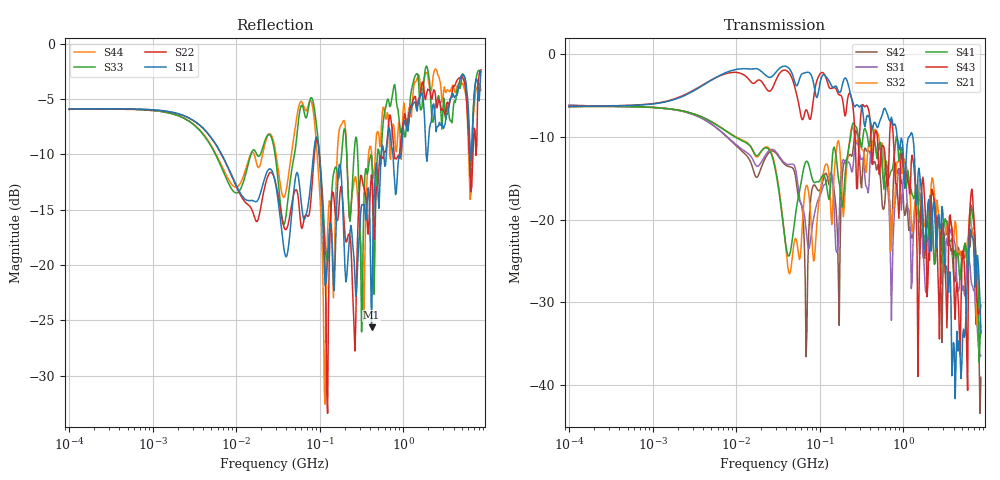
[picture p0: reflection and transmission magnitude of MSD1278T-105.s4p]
# MHz S MA R 50
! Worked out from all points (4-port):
!   498 points, 100 kHz to 8.5 GHz, reference 50 ohm
!   strongest paths, dB at 100 kHz, 1.698 MHz, 29.49 MHz, 500.7 MHz, 8.5 GHz:
!     S21: -6.3, -5.6, -2.3, -8.8, -33.7
!     S43: -6.3, -5.5, -3.3, -11.8, -30.4
!     S41: -6.4, -6.7, -14.0, -11.9, -33.4
!     S32: -6.4, -6.7, -13.7, -9.6, -32.9
!     S31: -6.2, -6.7, -11.7, -12.0, -36.4
!     S42: -6.2, -6.7, -11.9, -13.3, -39.1
!   lowest |S11| = -25.6 dB at 417.1 MHz (marker M1), VSWR 1.11, Z = 55.5 + j0.687 ohm
!   |S11| at or under -10 dB: 6.726 MHz to 84.3 MHz (77.58 MHz wide, 170 % of centre); 98.74 MHz to 546.1 MHz (447.3 MHz wide, 139 % of centre); 752.1 MHz to 938.7 MHz (186.6 MHz wide, 22.1 % of centre)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
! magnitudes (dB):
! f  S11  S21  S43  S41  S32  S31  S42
! 100 kHz  -5.9  -6.3  -6.3  -6.4  -6.4  -6.2  -6.2
! 68.65 MHz  -15.5  -2.2  -6.7  -13.0  -15.9  -21.2  -36.6
! 113.5 MHz  -20.3  -2.5  -2.4  -14.7  -13.8  -15.8  -14.7
! 417.1 MHz  -25.6  -8.8  -11.7  -8.9  -11.9  -10.8  -12.7
! 4 GHz  -4.7  -34.9  -24.6  -24.7  -22.4  -22.2  -26.6
! 6.612 GHz  -9.7  -22.1  -16.3  -18.6  -21.5  -27.9  -21.0
! 8.5 GHz  -2.5  -33.7  -30.4  -33.4  -32.9  -36.4  -39.1
